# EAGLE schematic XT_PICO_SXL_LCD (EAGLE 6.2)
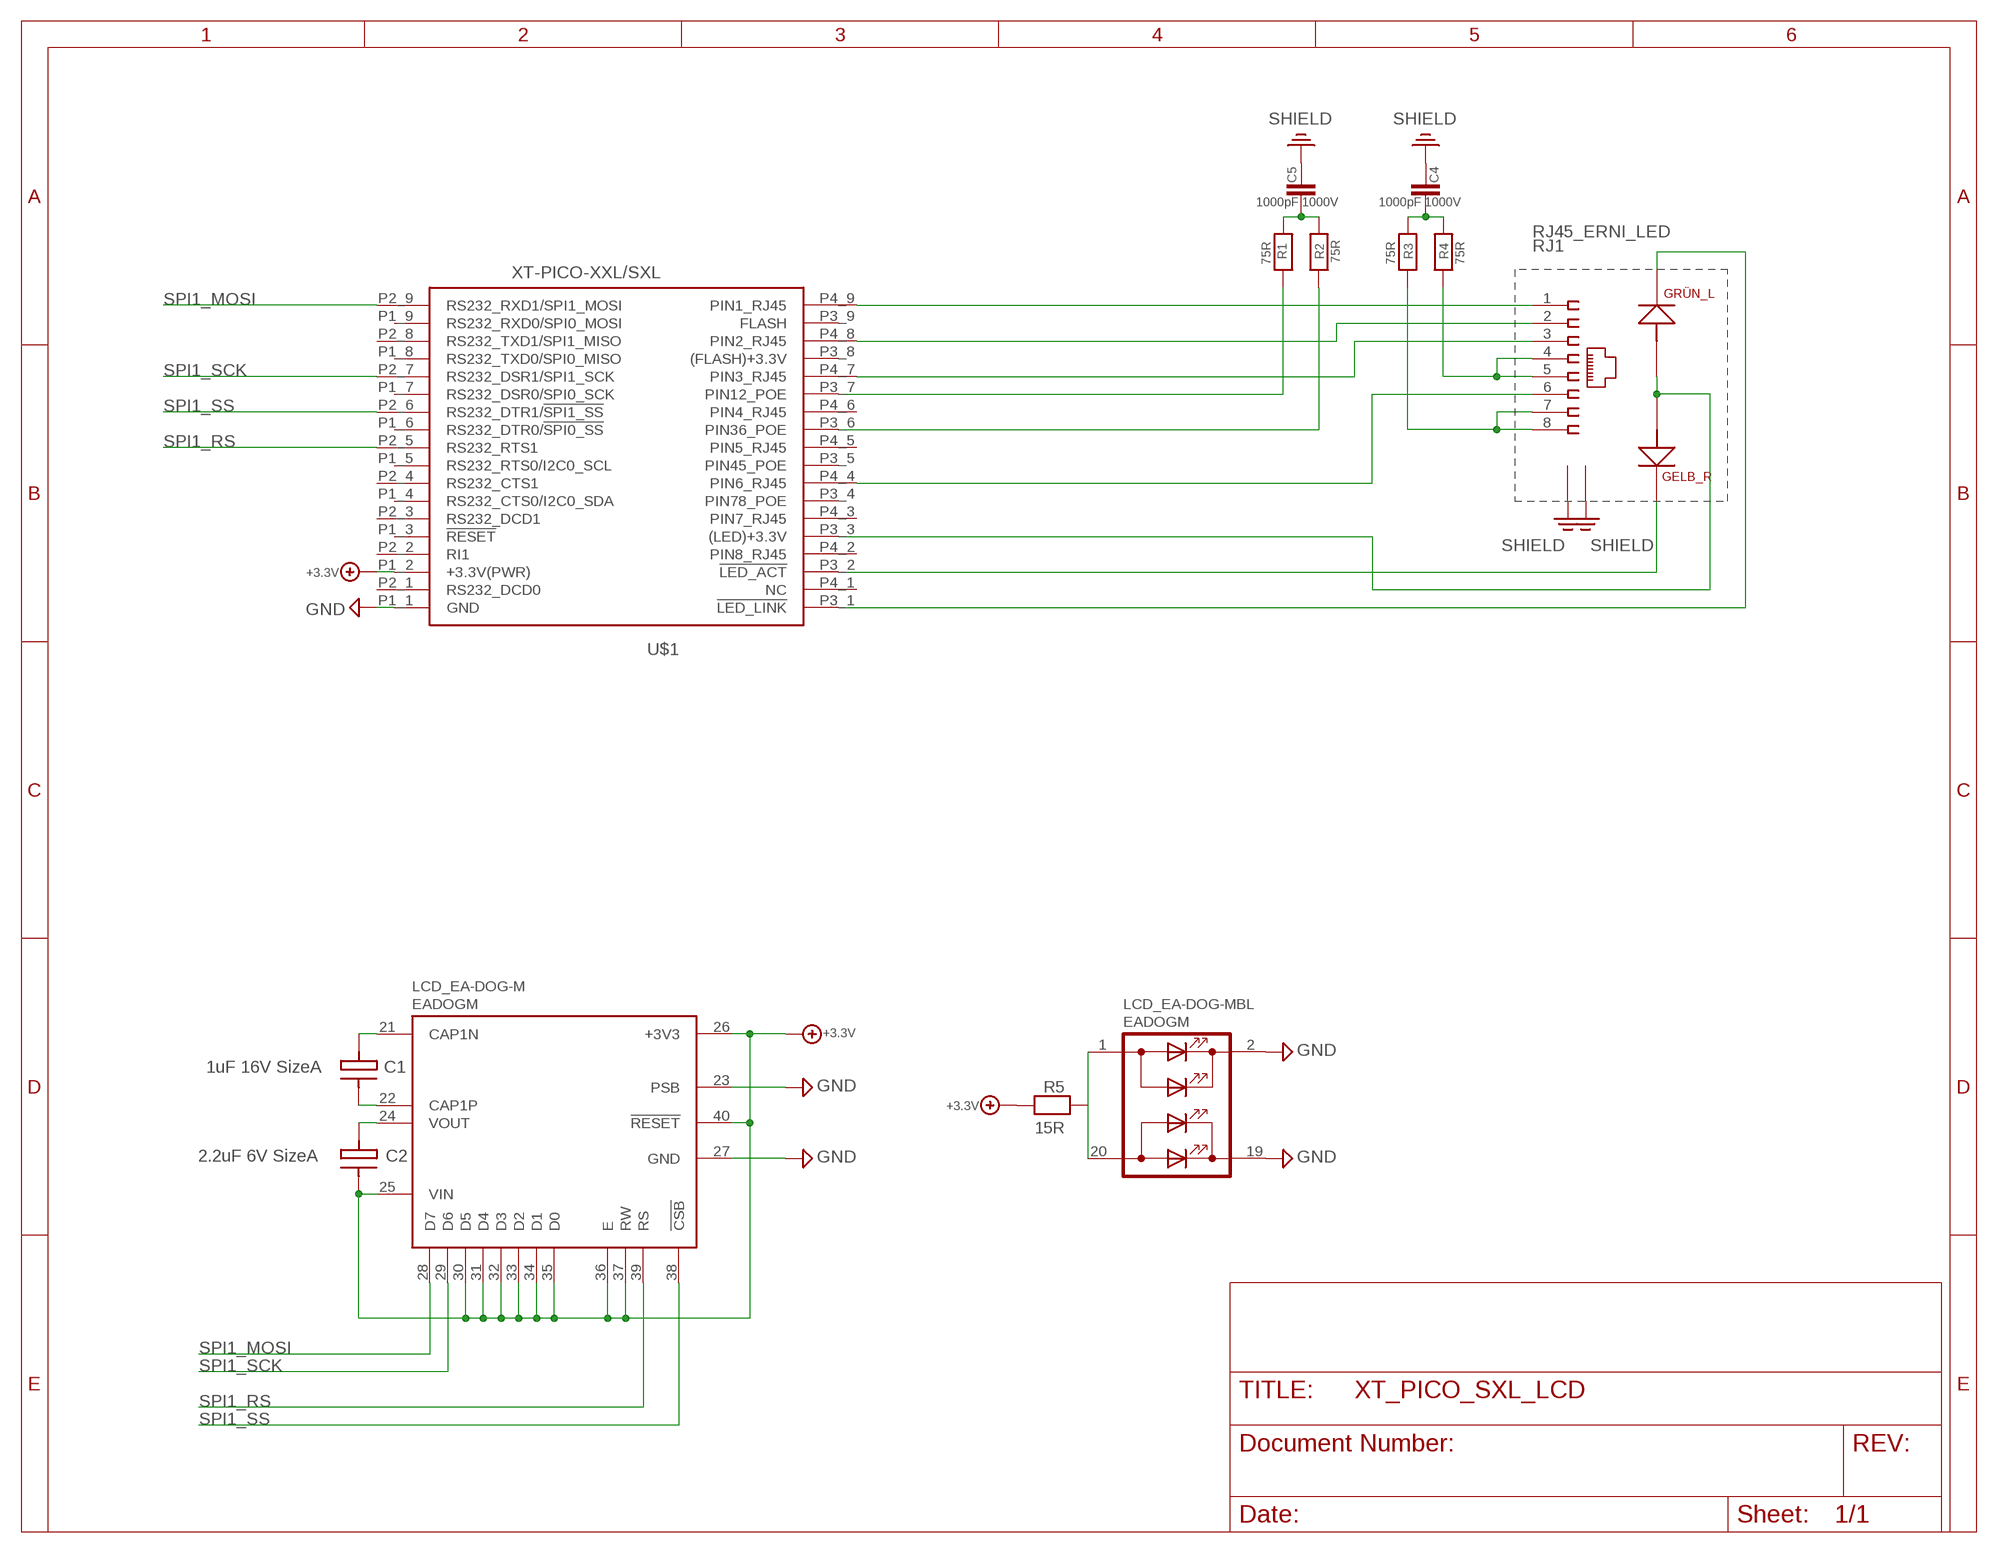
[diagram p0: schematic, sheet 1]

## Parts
C1  1uF 16V SizeA  C3216  [ORCAD_X_CT3216]
C2  2.2uF 6V SizeA  C3216  [ORCAD_X_CT3216]
C4  1000pF 1000V  CHIP-C-1210  [SMD-1210]
C5  1000pF 1000V  CHIP-C-1210  [SMD-1210]
LCD_EA-DOG-M  EADOGM  [EADOGM]
R1  75R  CHIP-R-0603  [SMD-0603]
R2  75R  CHIP-R-0603  [SMD-0603]
R3  75R  CHIP-R-0603  [SMD-0603]
R4  75R  CHIP-R-0603  [SMD-0603]
R5  15R  CHIP-R-0603  [SMD-0603@1]
RJ1  RJ45_ERNI_LED  [ORCAD_X_ERNI_RJ45_LED]
U$1  XT-PICO-XXL/SXL  [XT-PICO-XXL/SXL]

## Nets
+3.3V: C2.2(C-) LCD_EA-DOG-M.25(VIN) LCD_EA-DOG-M.26(+3V3) LCD_EA-DOG-M.30(D5) LCD_EA-DOG-M.31(D4) LCD_EA-DOG-M.32(D3) LCD_EA-DOG-M.33(D2) LCD_EA-DOG-M.34(D1) LCD_EA-DOG-M.35(D0) LCD_EA-DOG-M.36(E) LCD_EA-DOG-M.37(RW) LCD_EA-DOG-M.40(!RESET) R5.1 U$1.P1_2(+3.3V(PWR))
GND: LCD_EA-DOG-M.2(C1) LCD_EA-DOG-M.19(C2) LCD_EA-DOG-M.23(PSB) LCD_EA-DOG-M.27(GND) U$1.P1_1(GND)
N$1: RJ1.1 U$1.P4_9(PIN1_RJ45)
N$2: RJ1.3 U$1.P4_7(PIN3_RJ45)
N$3: R4.2 RJ1.4 RJ1.5
N$4: R1.2 U$1.P3_7(PIN12_POE)
N$5: LCD_EA-DOG-M.1(A1) LCD_EA-DOG-M.20(A2) R5.2
N$6: R2.2 U$1.P3_6(PIN36_POE)
N$7: C2.1(C+) LCD_EA-DOG-M.24(VOUT)
N$8: RJ1.2 U$1.P4_8(PIN2_RJ45)
N$9: C1.2(C-) LCD_EA-DOG-M.22(CAP1P)
N$10: R3.2 RJ1.7 RJ1.8
N$11: C1.1(C+) LCD_EA-DOG-M.21(CAP1N)
N$12: RJ1.6 U$1.P4_4(PIN6_RJ45)
N$15: RJ1.A1 RJ1.A2 U$1.P3_3((LED)+3.3V)
N$16: RJ1.K1 U$1.P3_2(!LED_ACT)
N$17: RJ1.K2 U$1.P3_1(!LED_LINK)
N$19: C4.2 R3.1 R4.1
N$20: C5.1 R1.1 R2.1
PE: RJ1.9 RJ1.10 ; supply symbol labelled SHIELD
SHIELD: C4.1 C5.2
SPI1_MOSI: LCD_EA-DOG-M.28(D7) U$1.P2_9(RS232_RXD1/SPI1_MOSI)
SPI1_RS: LCD_EA-DOG-M.39(RS) U$1.P2_5(RS232_RTS1)
SPI1_SCK: LCD_EA-DOG-M.29(D6) U$1.P2_7(RS232_DSR1/SPI1_SCK)
SPI1_SS: LCD_EA-DOG-M.38(!CSB) U$1.P2_6(RS232_DTR1/!SPI1_SS!)
Unconnected: U$1.P1_3(!RESET) U$1.P1_4(RS232_CTS0/I2C0_SDA) U$1.P1_5(RS232_RTS0/I2C0_SCL) U$1.P1_6(RS232_DTR0/!SPI0_SS!) U$1.P1_7(RS232_DSR0/SPI0_SCK) U$1.P1_8(RS232_TXD0/SPI0_MISO) U$1.P1_9(RS232_RXD0/SPI0_MOSI) U$1.P2_1(RS232_DCD0) U$1.P2_2(RI1) U$1.P2_3(RS232_DCD1) U$1.P2_4(RS232_CTS1) U$1.P2_8(RS232_TXD1/SPI1_MISO) U$1.P3_4(PIN78_POE) U$1.P3_5(PIN45_POE) U$1.P3_8((FLASH)+3.3V) U$1.P3_9(FLASH) U$1.P4_1(NC) U$1.P4_2(PIN8_RJ45) U$1.P4_3(PIN7_RJ45) U$1.P4_5(PIN5_RJ45) U$1.P4_6(PIN4_RJ45)

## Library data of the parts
C1 C2 = XTMACRO:C3216
C4 C5 = XTMACRO:CHIP-C-?: Chip capacitance
LCD_EA-DOG-M = XTMACRO:EADOGM: THT EA LCD Display With LED Backlight
R1-R4 = XTMACRO:CHIP-R-?: Chip resistors
R5 = mea-lib:CHIP-R-?: Chip resistors
RJ1 = XTMACRO:RJ45_ERNI_LED
U$1 = ak-devices:XT-PICO-XXL/SXL: AK-NORD XT-PICO-XXL/SXL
